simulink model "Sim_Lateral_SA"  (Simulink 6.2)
settings: Solver=ode45  StartTime=0.0  StopTime=50  RelTol=1e-3
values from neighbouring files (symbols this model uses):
  d2r = pi/180    (= 0.0174532925199)    [run.m]
  klr = [0.82083770557  -0.70145835124   0.75722294555   0.32691190448   0.14993771995;        0.55253708187   0.66141640307  -0.4963339086    0.20601876795  -0.07844376733]    [run.m]
  kls = [0.23009875115  -1.3857134134    0.5565800989    0.03843893525  0.1360972015;        0.22658853965   0.3268097242   -0.0904376422    0.0272194403  -0.00768778705]    [run.m]
  r2d = 180/pi    (= 57.2957795131)    [Pl.m]    (also in run.m)
undefined symbols (not defined in the file or in its folder): Alv, Blv, Clv, Dlv, KJmix, KSmix

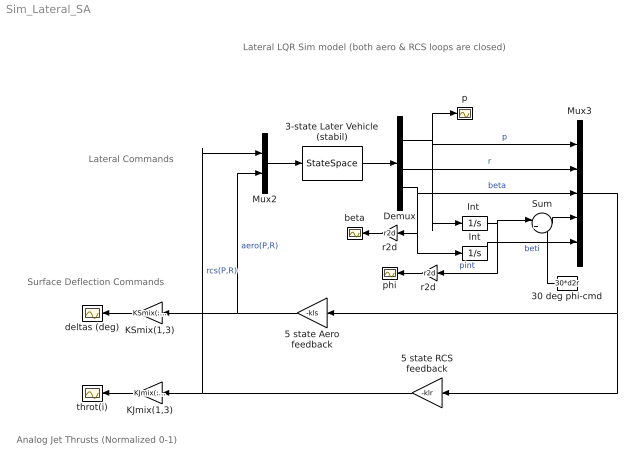
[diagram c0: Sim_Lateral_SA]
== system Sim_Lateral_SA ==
  note: Lateral LQR Sim model (both aero & RCS loops are closed)
  note: Lateral Commands
  note: Surface Deflection Commands
  note: Analog Jet Thrusts (Normalized 0-1)
  3-state Later Vehicle (stabil) : StateSpace  A=Alv  B=Blv  C=Clv  D=Dlv
  30 deg phi-cmd : Constant  Orientation=left  Value=30*d2r
  5 state Aero feedback : Gain  Orientation=left  Gain=-kls  Multiplication=Matrix(K*u)
  5 state RCS feedback : Gain  Orientation=left  Gain=-klr  Multiplication=Matrix(K*u)
  Demux : Demux  Outputs=3
  Int : Integrator
  "Int " : Integrator
  KJmix(1,3) : Gain  Orientation=left  Gain=KJmix(:,[1,3])  Multiplication=Matrix(K*u)
  KSmix(1,3) : Gain  Orientation=left  Gain=KSmix(:,[1,3])*r2d  Multiplication=Matrix(K*u)
  Mux2 : Mux  Inputs=[2,2]
  Mux3 : Mux  Inputs=5
  Sum : Sum  Inputs=|+-
  beta : Scope
  deltas (deg) : Scope
  p : Scope
  phi : Scope
  r2d : Gain  Orientation=left  Gain=r2d
  "r2d " : Gain  Orientation=left  Gain=r2d
  throt(i) : Scope
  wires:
  3-state Later Vehicle (stabil)/1 -> Demux/1
  Demux/1 -> Mux3/1, p/1, "Int "/1  "p"
  Demux/2 -> Mux3/2  "r"
  5 state RCS feedback/1 -> Mux2/1, KJmix(1,3)/1  "rcs(P,R)"
  Demux/3 -> Mux3/3, r2d/1, Int/1  "beta"
  5 state Aero feedback/1 -> Mux2/2, KSmix(1,3)/1  "aero(P,R)"
  KSmix(1,3)/1 -> deltas (deg)/1
  r2d/1 -> beta/1
  Mux3/1 -> 5 state RCS feedback/1, 5 state Aero feedback/1
  "Int "/1 -> Sum/1, "r2d "/1  "pint"
  30 deg phi-cmd/1 -> Sum/2
  Sum/1 -> Mux3/4
  Int/1 -> Mux3/5  "beti"
  "r2d "/1 -> phi/1
  KJmix(1,3)/1 -> throt(i)/1
  Mux2/1 -> 3-state Later Vehicle (stabil)/1
